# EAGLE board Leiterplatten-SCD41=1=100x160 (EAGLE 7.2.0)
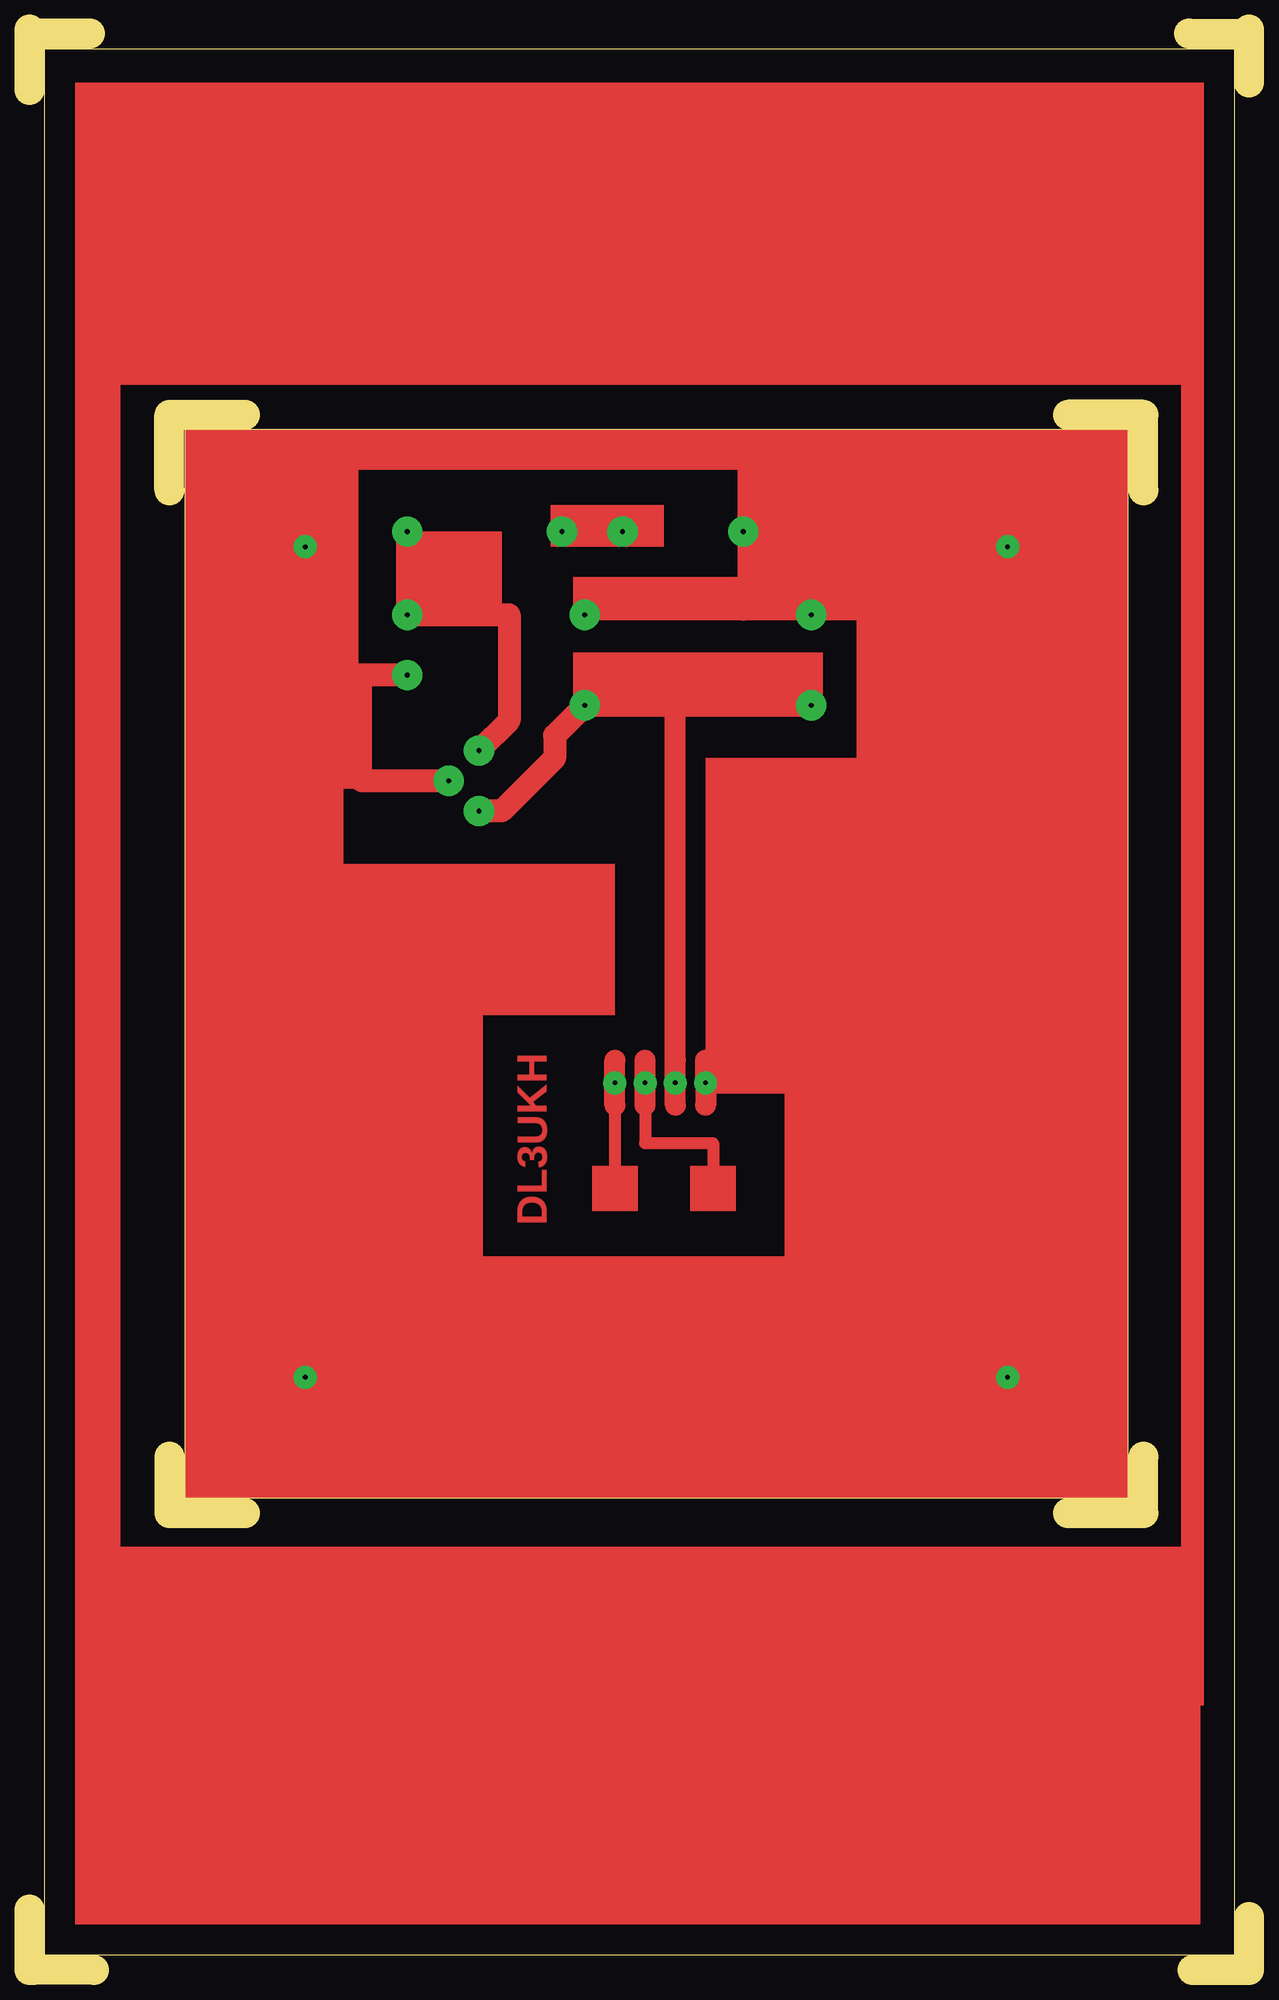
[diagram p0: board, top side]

Size 102.55 x 163.2 mm. Coordinates in mm from the lower left corner, seen from the top.
Outline: 5.4,0 0.32,0
Outline: 0,0 0,5.08
Outline: 97.79,0 102.55,0 102.55,4.45
Outline: 5.08,162.88 0,162.88
Outline: 0,158.12 0,162.88
Outline: 0,162.88 0,163.2
Outline: 102.55,158.75 102.55,163.2
Outline: 97.47,162.88 102.23,162.88
Outline: 11.75,124.46 11.75,130.81 18.1,130.81
Outline: 11.75,43.18 11.75,38.42 18.1,38.42
Outline: 87.31,38.42 93.66,38.42 93.66,43.18
Outline: 93.66,124.46 93.66,130.81 87.31,130.81
Outline: 1.27,1.27 101.28,1.27 101.28,161.61 1.27,161.61 1.27,1.27
Outline: 13.02,129.54 13.02,39.69 92.39,39.69 92.39,129.54 13.02,129.54
Copper layers (1*16): Top 0.035mm / dielectric 1.5mm / Bottom 0.035mm
Design rules "default": minimum track width 10mil, minimum drill 24mil, track to track 8mil, track to pad 8mil, pad to pad 8mil, via to via 8mil, smd to smd 8mil, copper to edge 40mil, drill to drill 8mil, minimum pad ring 10mil, minimum via ring 8mil, stop-mask expansion 4mil, vias tented up to drill 0mil, thermal gap 10mil

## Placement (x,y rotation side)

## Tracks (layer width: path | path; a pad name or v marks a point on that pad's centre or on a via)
S$1  (via drill 0.4 pad 1.93)
  other vias: 54.29,74.61
S$2  (via drill 0.4 pad 1.93)
  Top 1.016: v51.75,74.61 51.75,69.53 57.47,69.53 57.47,65.72
S$3  (via drill 0.4 pad 2.54)
  Top 1.93: v49.85,120.97 v44.77,120.97
S$4  (via drill 0.4 pad 1.93)
  Top 1.016: v49.21,74.61 49.21,65.72
S$5  (via drill 0.4 pad 2.54)
  Top 1.93: v31.75,120.97 v31.75,113.98 40.32,113.98 40.32,105.09 v37.78,102.55
S$6  (via drill 0.4 pad 1.93)
  Top 1.016: 73.34,74.61 73.34,64.45
  Top 1.778: v56.83,74.61 56.83,72.71 | v56.83,74.61 56.83,76.52 | 54.29,72.71 54.29,76.52 54.29,107.31 | 51.75,72.71 51.75,76.52 | 49.21,72.71 49.21,76.52 | v56.83,74.61 73.34,74.61
S$7  (via drill 0.4 pad 2.54)
  Top 1.93: v37.78,97.47 39.69,97.47 44.13,101.92 44.13,103.82 v46.67,106.36 v65.72,106.36
S$8  (via drill 0.4 pad 1.93)
  other vias: 82.23,49.85
S$9  (via drill 0.4 pad 1.93)
  other vias: 82.23,119.7
S$10  (via drill 0.4 pad 2.54)
  Top 1.016: 73.66,71.44 80.96,71.44 80.96,113.98 73.34,113.98 | v31.75,108.9 28.26,108.9 | 28.26,108.9 28.26,100.01 34.93,100.01 v35.24,100.01 | 28.26,108.9 27.3,108.9 23.18,108.9 | 23.18,108.9 23.18,126.68 60.01,126.68 v60.01,120.97 60.01,113.98 | 60.01,113.98 v65.72,113.98 73.34,113.98 | 60.01,113.98 v46.67,113.98 | 23.18,108.9 15.24,108.9 15.24,41.59 68.9,41.59 | 73.34,71.75 73.34,113.98
  Top 1.93: 34.93,100.01 27.94,100.01 | v31.75,108.9 27.3,108.9
S$29  (via drill 0.4 pad 1.93)
  other vias: 23.18,49.85
S$34  (via drill 0.4 pad 1.93)
  other vias: 23.18,119.7
(copper drawn outside any net)
  shapes: Top area x37

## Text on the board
Top: DL3UKH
